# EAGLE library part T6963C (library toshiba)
DOT MATRIX LCD CONTROL LSI Source: LCD Microcontroller Datasheet - Toshiba T6963C.pdf
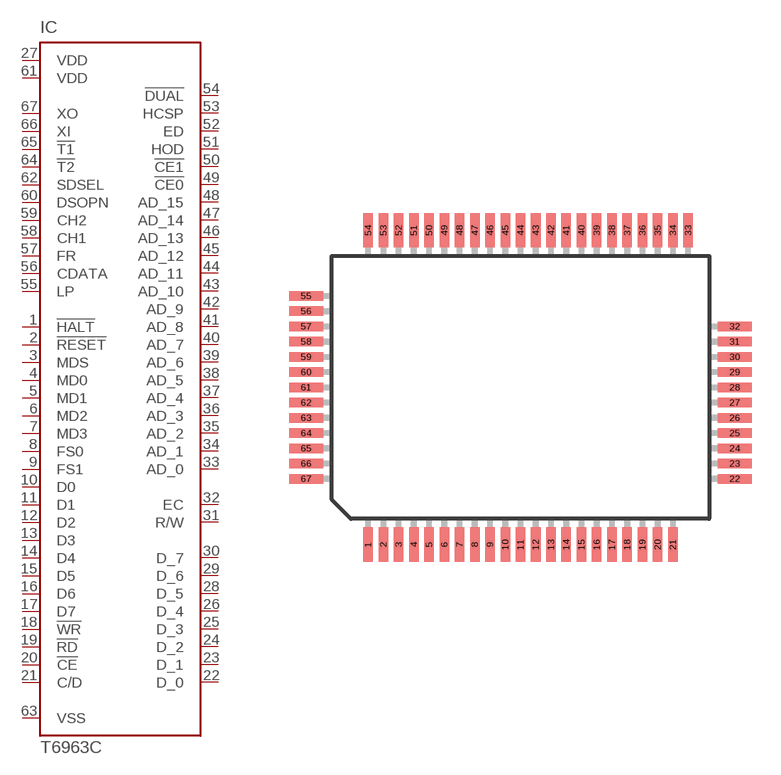
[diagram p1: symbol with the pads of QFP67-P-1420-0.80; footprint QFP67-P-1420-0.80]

Designator prefix IC

## T6963C (OC_FARNELL: unknown; OC_NEWARK: unknown)  [QFP67-P-1420-0.80]
1  !HALT  in
2  !RESET  in
3  MDS  in
4  MD0  in
5  MD1  in
6  MD2  in
7  MD3  in
8  FS0  in
9  FS1  in
10  D0  in
11  D1  in
12  D2  in
13  D3  in
14  D4  in
15  D5  in
16  D6  in
17  D7  in
18  !WR  in
19  !RD  in
20  !CE  in
21  C/D  in
22  D_0  in
23  D_1  in
24  D_2  in
25  D_3  in
26  D_4  in
27  VDD  out
28  D_5  in
29  D_6  in
30  D_7  in
31  R/W  in
32  EC  in
33  AD_0  in
34  AD_1  in
35  AD_2  in
36  AD_3  in
37  AD_4  in
38  AD_5  in
39  AD_6  in
40  AD_7  in
41  AD_8  in
42  AD_9  in
43  AD_10  in
44  AD_11  in
45  AD_12  in
46  AD_13  in
47  AD_14  in
48  AD_15  in
49  !CE0  in
50  !CE1  in
51  HOD  in
52  ED  in
53  HCSP  in
54  !DUAL  in
55  LP  in
56  CDATA  in
57  FR  in
58  CH1  in
59  CH2  in
60  DSOPN  in
61  VDD  out
62  SDSEL  in
63  VSS  out
64  !T2  in
65  !T1  in
66  XI  in
67  XO  out

## Footprint QFP67-P-1420-0.80 (pad centres in mm)
QFP76-P-1420-0.80 Source: LCD Microcontroller Datasheet - Toshiba T6963C.pdf
smd 0.5 x 1.8: 1 -8,-8.25; 2 -7.2,-8.25; 3 -6.4,-8.25; 4 -5.6,-8.25; 5 -4.8,-8.25; 6 -4,-8.25; 7 -3.2,-8.25; 8 -2.4,-8.25; 9 -1.6,-8.25; 10 -0.8,-8.25; 11 0,-8.25; 12 0.8,-8.25; 13 1.6,-8.25; 14 2.4,-8.25; 15 3.2,-8.25; 16 4,-8.25; 17 4.8,-8.25; 18 5.6,-8.25; 19 6.4,-8.25; 20 7.2,-8.25; 21 8,-8.25; 33 8.8,8.25; 34 8,8.25; 35 7.2,8.25; 36 6.4,8.25; 37 5.6,8.25; 38 4.8,8.25; 39 4,8.25; 40 3.2,8.25; 41 2.4,8.25; 42 1.6,8.25; 43 0.8,8.25; 44 0,8.25; 45 -0.8,8.25; 46 -1.6,8.25; 47 -2.4,8.25; 48 -3.2,8.25; 49 -4,8.25; 50 -4.8,8.25; 51 -5.6,8.25; 52 -6.4,8.25; 53 -7.2,8.25; 54 -8,8.25
smd 1.8 x 0.5: 22 11.25,-4.8; 23 11.25,-4; 24 11.25,-3.2; 25 11.25,-2.4; 26 11.25,-1.6; 27 11.25,-0.8; 28 11.25,0; 29 11.25,0.8; 30 11.25,1.6; 31 11.25,2.4; 32 11.25,3.2; 55 -11.25,4.8; 56 -11.25,4; 57 -11.25,3.2; 58 -11.25,2.4; 59 -11.25,1.6; 60 -11.25,0.8; 61 -11.25,0; 62 -11.25,-0.8; 63 -11.25,-1.6; 64 -11.25,-2.4; 65 -11.25,-3.2; 66 -11.25,-4; 67 -11.25,-4.8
